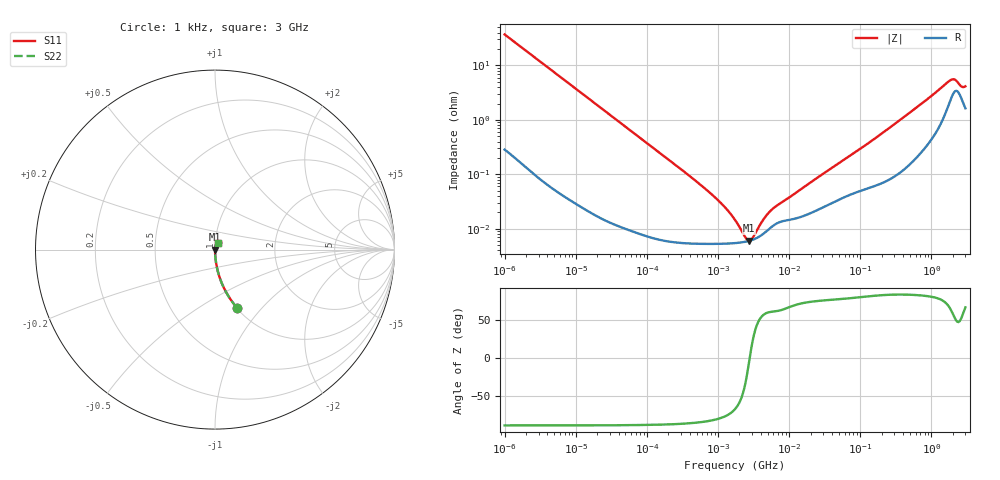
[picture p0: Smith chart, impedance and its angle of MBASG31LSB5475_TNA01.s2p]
! MBASG31LSB5475_TNA01  S-PARAMETER MODEL  ( Standard Model )
! Model Generated by TAIYO YUDEN Corporation (http://www.ty-top.com)
! Version 1.0
! TAIYO YUDEN Control No. 220601
! Copyright(c) 2012 TAIYO YUDEN CO.,LTD. All Rights Reserved.
! Product Description (link to TY-COMPAS)
! https://ds.yuden.co.jp/TYCOMPAS/or/detail?pn=MBASG31LSB5475KTNA01&u=M
! Products Name : Multilayer Ceramic Capacitors
! Characteristics :
!  Capacitance : 4.7 [uF] , Rated Voltage : 35 [V] , TCC : X5R
!  Case Size : 3.2 x 1.6 / 0.126 x 0.063 [mm/inch] , Thickness : 1.6 / 0.063 [mm/inch]
!  (Conditions: Temperature = 25 [degC] , DC Bias Voltage = 0 [V])
! External Node Assignments :
!  1  o---| |---o  2
! GND o---------o GND
! Frequency Range : 1kHz  -  3GHz  [ 401 STEP ]
# MHZ S RI R 50
! Freq[MHz].  S11 Real  S11 Imag  S21 Real  S21 Imag  S12 Real  S12 Imag  S22 Real  S22 Imag
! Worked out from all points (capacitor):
!   401 points, 1 kHz to 3 GHz, reference 50 ohm
!   read as one part in series: C = 4.29 uF near 1.077 kHz
!   lowest |Z| = 6.04 mohm at 2.709 MHz (marker M1)
!   series resonance near 2.79 MHz, so ESL is about 760 pH
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0.001  0.1225 -0.324  0.8775 0.324  0.8775 0.324  0.1225 -0.324
0.001685  0.0477 -0.2095  0.9523 0.2095  0.9523 0.2095  0.0477 -0.2095
0.00306  0.0154 -0.1197  0.9846 0.1197  0.9846 0.1197  0.0154 -0.1197
0.005768  0.00462 -0.0644  0.9954 0.0644  0.9954 0.0644  0.00462 -0.0644
0.01216  0.00119 -0.0307  0.9988 0.0307  0.9988 0.0307  0.00119 -0.0307
0.147855  6.97e-05 -0.00255  0.9999 0.00255  0.9999 0.00255  6.97e-05 -0.00255
0.821683  5.3e-05 -0.000422  0.9999 0.000422  0.9999 0.000422  5.3e-05 -0.000422
1.238299  5.34e-05 -0.000247  0.9999 0.000247  0.9999 0.000247  5.34e-05 -0.000247
1.732051  5.47e-05 -0.000135  0.9999 0.000135  0.9999 0.000135  5.47e-05 -0.000135
2.087011  5.61e-05 -8.07e-05  0.9999 8.07e-05  0.9999 8.07e-05  5.61e-05 -8.07e-05
2.709407  5.99e-05 -8.07e-06  0.9999 8.07e-06  0.9999 8.07e-06  5.99e-05 -8.07e-06
3.517417  6.8e-05 6.43e-05  0.9999 -6.43e-05  0.9999 -6.43e-05  6.8e-05 6.43e-05
3.789741  7.18e-05 8.54e-05  0.9999 -8.54e-05  0.9999 -8.54e-05  7.18e-05 8.54e-05
4.919932  9.27e-05 0.000159  0.9999 -0.000159  0.9999 -0.000159  9.27e-05 0.000159
5.928204  0.000113 0.000207  0.9999 -0.000207  0.9999 -0.000207  0.000113 0.000207
21.06097  0.0002 0.000719  0.9998 -0.000719  0.9998 -0.000719  0.0002 0.000719
104.6572  0.000515 0.00303  0.9995 -0.00303  0.9995 -0.00303  0.000515 0.00303
256.0921  0.000852 0.00707  0.9991 -0.00707  0.9991 -0.00707  0.000852 0.00707
1847.629  0.0246 0.0462  0.9754 -0.0462  0.9754 -0.0462  0.0246 0.0462
2066.299  0.0326 0.0429  0.9674 -0.0429  0.9674 -0.0429  0.0326 0.0429
2682.519  0.0239 0.0315  0.9761 -0.0315  0.9761 -0.0315  0.0239 0.0315
3000  0.0174 0.0368  0.9826 -0.0368  0.9826 -0.0368  0.0174 0.0368
